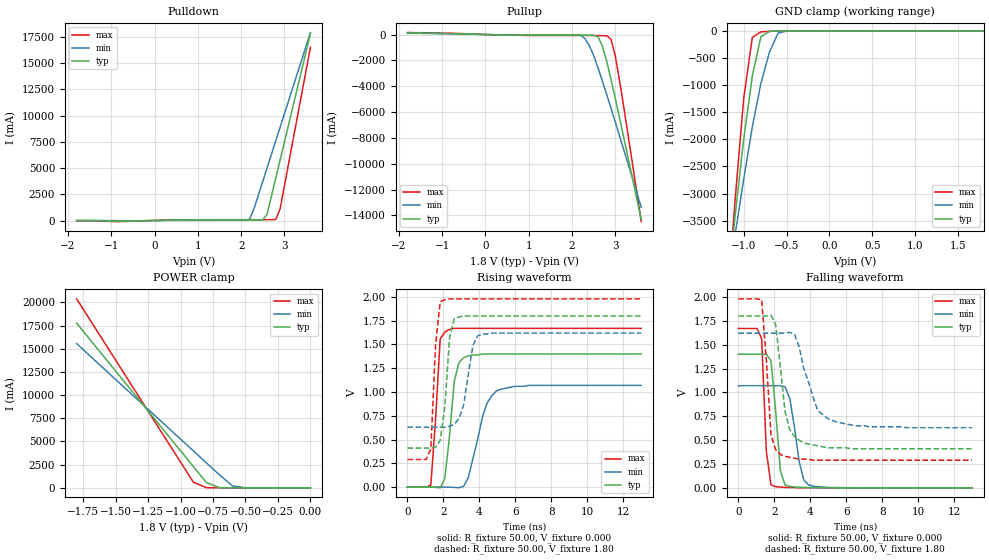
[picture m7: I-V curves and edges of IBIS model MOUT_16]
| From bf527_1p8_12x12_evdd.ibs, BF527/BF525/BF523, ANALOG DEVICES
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|   Model prw1216cdg_25
[Model]   MOUT_16
Model_type   I/O
Polarity   Non-Inverting
Enable   Active-Low
Vinl =   0.70V
Vinh =   1.00V
Vmeas =   1.20V
Cref =  50.00pF
Rref =   1.00M
Vref =  0.000V
C_comp   4.56pF   4.11pF   5.02pF
[Temperature Range]   25.00   0.12k   -40.00
[Voltage Range]   1.80V   1.62V   1.98V
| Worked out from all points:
|   slope of the pulldown table from 0 to 0.27 V, typ, clamps not added: 13.6 ohm
|   slope of the pullup table from 0 to 0.27 V, typ, clamps not added: 13.3 ohm
|   GND clamp passes 1 mA (typ) near -0.53 V on its own axis
|   POWER clamp passes 1 mA (typ) near -0.53 V on its own axis
|   rising waveform, R_fixture 50.00, V_fixture 0.000: 20-80 % time 424ps typ, 849ps min, 333ps max; typ from 0 V to 1.4 V
|   rising waveform, R_fixture 50.00, V_fixture 1.80: 20-80 % time 360ps typ, 522ps min, 292ps max; typ from 0.41 V to 1.8 V
|   falling waveform, R_fixture 50.00, V_fixture 0.000: 20-80 % time 375ps typ, 535ps min, 245ps max; typ from 1.4 V to 0 V
|   falling waveform, R_fixture 50.00, V_fixture 1.80: 20-80 % time 565ps typ, 941ps min, 359ps max; typ from 1.8 V to 0.41 V
[Pulldown]
| voltage   I(typ)   I(min)   I(max)
-1.8V     -10mA      0A         -10mA
-900mV    -54mA      -13mA      -100mA
600mV     35.42mA    19.27mA    58.01mA
2.1V      42.7mA     29mA       73.65mA
2.2V      42.77mA    140mA      73.7mA
2.3V      43.22mA    1.16A      73.75mA
2.5V      59.87mA    3.73A      74.66mA
2.6V      610mA      5.02A      77.37mA
2.8V      4.04A      7.6A       99.23mA
2.9V      5.76A      8.88A      1.1A
3.6V      17.81A     17.91A     16.5A
[Pullup]
| voltage   I(typ)   I(min)   I(max)
-1.8V     130mA      100mA      150mA
2.2V      -46.27mA   -53.72mA   -75.17mA
2.3V      -46.79mA   -320mA     -75.36mA
2.4V      -49mA      -860mA     -75.6mA
2.5V      -56.4mA    -1.62A     -76.56mA
2.6V      -160mA     -2.56A     -80.35mA
2.7V      -870mA     -3.57A     -87.33mA
2.8V      -2.04A     -4.62A     -98.53mA
2.9V      -3.45A     -5.69A     -350mA
3V        -4.95A     -6.77A     -1.65A
3.1V      -6.48A     -7.86A     -3.58A
3.6V      -14.33A    -13.37A    -14.48A
[GND_clamp]
| voltage   I(typ)   I(min)   I(max)
-1.8V     -14.28A    -11.35A    -18.41A
-1.2V     -4.9A      -4.81A     -5.19A
-1.1V     -3.4A      -3.75A     -3.1A
-1V       -1.99A     -2.73A     -1.24A
-900mV    -830mA     -1.77A     -120mA
-800mV    -110mA     -970mA     -19.15mA
-700mV    -9.85mA    -390mA     -9.73mA
-600mV    -2.55mA    -42.82mA   -3.48mA
-500mV    -450uA     -4.35mA    -550uA
1.8V      150pA      1.58uA     73.18pA
[POWER_clamp]
| voltage   I(typ)   I(min)   I(max)
-1.8V     17.76A     15.56A     20.38A
-900mV    2.28A      3.97A      590mA
-800mV    570mA      2.68A      16.99mA
-700mV    17.03mA    1.4A       7.08mA
-600mV    2.36mA     210mA      2.77mA
-500mV    460uA      11.86mA    530uA
0V        150pA      7.78nA     85.42pA
[Ramp]
| variable   typ   min   max
dV/dt_r   0.84/0.38n   0.64/0.75n   1.00/0.22n
dV/dt_f   0.83/0.50n   0.59/0.86n   1.01/0.27n
R_load = 50.00
[Rising Waveform]
R_fixture = 50.00
V_fixture = 0.000
V_fixture_min = 0.000
V_fixture_max = 0.000
L_fixture = 0.000H
C_fixture = 0.000F
| time   V(typ)   V(min)   V(max)
0s        0V         0V         0V
1.3ns     -330uV     54.08uV    22.3mV
1.56ns    -2.53mV    42.27uV    700mV
1.82ns    -8.14mV    -27.05uV   1.56V
2.08ns    92.1mV     -360uV     1.63V
2.6ns     1.11V      -3.18mV    1.67V
3.12ns    1.36V      7.77mV     1.67V
4.42ns    1.4V       880mV      1.67V
4.94ns    1.4V       1.01V      1.67V
13ns      1.4V       1.07V      1.67V
[Rising Waveform]
R_fixture = 50.00
V_fixture = 1.80
V_fixture_min = 1.62
V_fixture_max = 1.98
L_fixture = 0.000H
C_fixture = 0.000F
| time   V(typ)   V(min)   V(max)
0s        410mV      630mV      290mV
1.3ns     410mV      630mV      400mV
1.56ns    420mV      630mV      1.49V
1.82ns    490mV      630mV      1.95V
2.08ns    850mV      630mV      1.97V
2.34ns    1.57V      640mV      1.98V
2.6ns     1.77V      660mV      1.98V
3.12ns    1.8V       860mV      1.98V
3.9ns     1.8V       1.59V      1.98V
13ns      1.8V       1.62V      1.98V
[Falling Waveform]
R_fixture = 50.00
V_fixture = 0.000
V_fixture_min = 0.000
V_fixture_max = 0.000
L_fixture = 0.000H
C_fixture = 0.000F
| time   V(typ)   V(min)   V(max)
0s        1.4V       1.07V      1.67V
1.3ns     1.4V       1.07V      1.56V
1.56ns    1.4V       1.07V      380mV
1.82ns    1.33V      1.07V      30.97mV
2.34ns    180mV      1.07V      7.49mV
2.6ns     30.57mV    1.06V      4.81mV
2.86ns    14.65mV    940mV      3.35mV
3.38ns    6.24mV     280mV      1.4mV
3.9ns     3.41mV     32.66mV    750uV
13ns      -28.62uV   -8.11uV    0V
[Falling Waveform]
R_fixture = 50.00
V_fixture = 1.80
V_fixture_min = 1.62
V_fixture_max = 1.98
L_fixture = 0.000H
C_fixture = 0.000F
| time   V(typ)   V(min)   V(max)
0s        1.8V       1.62V      1.98V
1.3ns     1.8V       1.62V      1.97V
1.82ns    1.81V      1.62V      550mV
2.08ns    1.71V      1.62V      400mV
2.34ns    1.26V      1.62V      350mV
2.86ns    610mV      1.63V      320mV
3.64ns    470mV      1.25V      300mV
4.42ns    440mV      810mV      290mV
5.46ns    420mV      690mV      290mV
13ns      410mV      630mV      290mV
